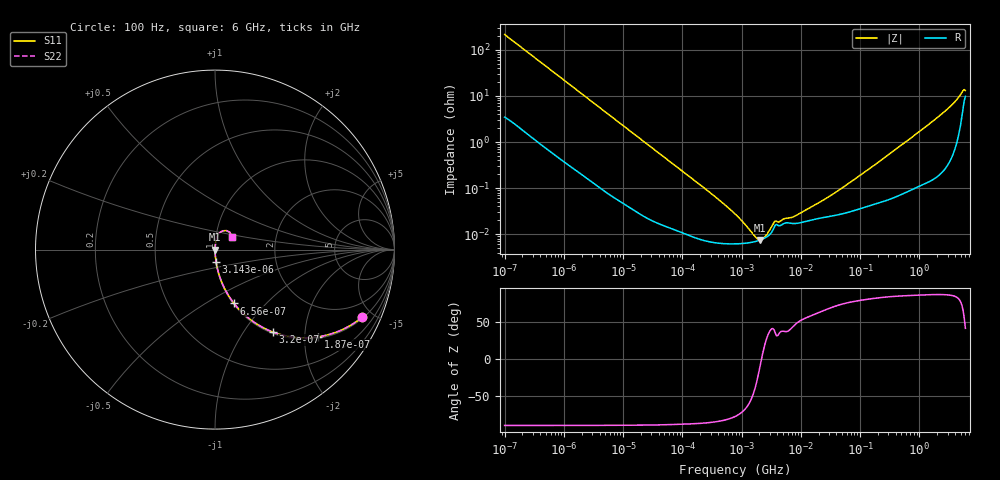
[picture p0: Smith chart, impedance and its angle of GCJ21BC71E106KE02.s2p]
!Murata Part Number: GCJ21BC71E106KE02
!These Parameters are Measured in Series Mode Connection
!Data Generated on Mar 13, 2026
!  o--ll--o
!Port1  Port2
!  o------o
!Operation Temp=25[degC], DC Bias Voltage=0[V]
!Freq. Start=100[Hz] Stop=6[GHz] 401[Steps]
# Hz S RI R 50
!Freq.(Hz) S11(Real) S11(Imag) S21(Real) S21(Imag) S12(Real) S12(Imag) S22(Real) S22(Imag)
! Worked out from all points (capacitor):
!   401 points, 100 Hz to 6 GHz, reference 50 ohm
!   read as one part in series: C = 7.32 uF near 109 Hz
!   lowest |Z| = 7.53 mohm at 2.074 MHz (marker M1)
!   series resonance near 2.166 MHz, so ESL is about 740 pH
!   S11 on the Smith chart (normalised r, x): 100 Hz: 1.07, -4.33; 187 Hz: 1.04, -2.33; 320 Hz: 1.02, -1.37; 656 Hz: 1.01, -0.67; 3.143 kHz: 1.00, -0.14; 6 GHz: 1.20, +0.17
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100  0.8202 -0.3761  0.1798 0.3761  0.1798 0.3761  0.8202 -0.3761
187  0.575 -0.4861  0.425 0.4861  0.425 0.4861  0.575 -0.4861
320  0.3223 -0.4592  0.6777 0.4592  0.6777 0.4592  0.3223 -0.4592
458  0.1917 -0.3855  0.8083 0.3855  0.8083 0.3855  0.1917 -0.3855
656  0.1061 -0.2997  0.8939 0.2997  0.8939 0.2997  0.1061 -0.2997
2008  0.0141 -0.1096  0.9859 0.1096  0.9859 0.1096  0.0141 -0.1096
3143  0.00635 -0.071  0.9936 0.071  0.9936 0.071  0.00635 -0.071
40335  0.0002 -0.00573  0.9998 0.00573  0.9998 0.00573  0.0002 -0.00573
302498  6.79e-05 -0.000772  0.9999 0.000772  0.9999 0.000772  6.79e-05 -0.000772
774597  6.16e-05 -0.000269  0.9999 0.000269  0.9999 0.000269  6.16e-05 -0.000269
1516199  6.69e-05 -8.07e-05  0.9999 8.07e-05  0.9999 8.07e-05  6.69e-05 -8.07e-05
2074311  7.47e-05 -9.7e-06  0.9999 9.7e-06  0.9999 9.7e-06  7.47e-05 -9.7e-06
2713602  8.88e-05 5.17e-05  0.9999 -5.17e-05  0.9999 -5.17e-05  8.88e-05 5.17e-05
3712478  0.000158 0.000111  0.9998 -0.000111  0.9998 -0.000111  0.000158 0.000111
7599586  0.00017 0.00017  0.9998 -0.00017  0.9998 -0.00017  0.00017 0.00017
1.555665e7  0.000205 0.000343  0.9998 -0.000343  0.9998 -0.000343  0.000205 0.000343
4.556224e7  0.000269 0.000893  0.9997 -0.000893  0.9997 -0.000893  0.000269 0.000893
3.124326e8  0.000597 0.00544  0.9994 -0.00544  0.9994 -0.00544  0.000597 0.00544
1.637704e9  0.00223 0.0273  0.9978 -0.0273  0.9978 -0.0273  0.00223 0.0273
3.666503e9  0.00953 0.0656  0.9905 -0.0656  0.9905 -0.0656  0.00953 0.0656
5.245841e9  0.0464 0.105  0.9536 -0.105  0.9536 -0.105  0.0464 0.105
6e9  0.0947 0.0716  0.9053 -0.0716  0.9053 -0.0716  0.0947 0.0716
